PROGRAM p06_detekcijaFronte
VAR
	S0: BOOL;
	S1: BOOL;
	L0: BOOL;
	L1: BOOL;
	L2: BOOL;
	PozitivnaFronta: R_TRIG;
	NegativnaFronta: F_TRIG;
	PozitivnaFrontaIzraz: R_TRIG;		
END_VAR

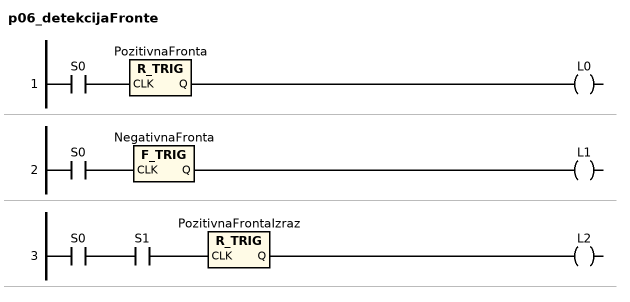
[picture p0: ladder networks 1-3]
// NETWORK 1
PozitivnaFronta(CLK := S0); // R_TRIG
L0 := PozitivnaFronta.Q;

// NETWORK 2
NegativnaFronta(CLK := S0); // F_TRIG
L1 := NegativnaFronta.Q;

// NETWORK 3
PozitivnaFrontaIzraz(CLK := S0 AND S1); // R_TRIG
L2 := PozitivnaFrontaIzraz.Q;

END_PROGRAM
